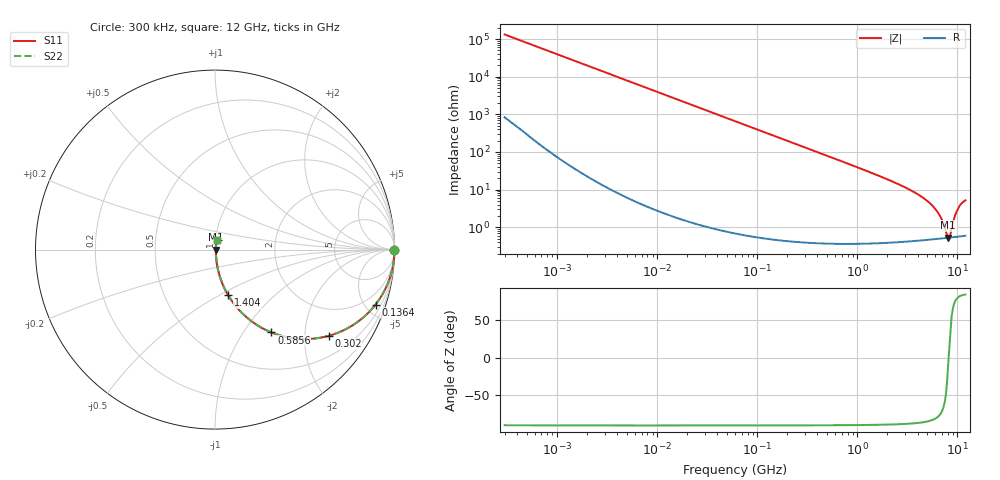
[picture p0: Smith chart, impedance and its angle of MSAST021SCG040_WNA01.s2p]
! MSAST021SCG040_WNA01  S-PARAMETER MODEL  ( General Type )
! Model Generated by TAIYO YUDEN Corporation (http://www.ty-top.com)
! Version 2.0
! TAIYO YUDEN Control No. 181101
! Copyright(c) 2015 TAIYO YUDEN CO.,LTD. All Rights Reserved.
! Product Description (link to TY-COMPAS)
! https://ds.yuden.co.jp/TYCOMPAS/or/detail?pn=MSAST021SCG040BWNA01&u=M
! Products Name : Multilayer Ceramic Capacitors
! Characteristics :
!  Capacitance : 4 pF , Rated Voltage : 25V , TCC : CG / C0G
!  Case Size : 0.25 x 0.125 / 0.0098 x 0.0049 [mm/inch] , Thickness : 0.125 / 0.0049 [mm/inch]
!  (Conditions: Temperature = 25 degC , DC Bias Current/Voltage = 0A / 0V)
! External Node Assignments :
!  1  o---| |---o  2
! GND o---------o GND
! Frequency Range : 0.3MHz  -  12000MHz  [ 401 STEP ]
# MHz S RI R 50
! Freq[MHz].  S11 Real  S11 Imag  S21 Real  S21 Imag  S12 Real  S12 Imag  S22 Real  S22 Imag
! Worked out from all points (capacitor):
!   401 points, 300 kHz to 12 GHz, reference 50 ohm
!   read as one part in series: C = 4 pF near 316.3 kHz
!   lowest |Z| = 534 mohm at 8.065 GHz (marker M1)
!   series resonance near 8.167 GHz, so ESL is about 95 pH
!   S11 on the Smith chart (normalised r, x): 300 kHz: open; 136.4 MHz: 1.01, -5.83; 302 MHz: 1.01, -2.63; 585.6 MHz: 1.01, -1.35; 1.404 GHz: 1.01, -0.55; 12 GHz: 1.01, +0.10
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0.3  1 -0.000754  5.31e-06 0.000754  5.31e-06 0.000754  1 -0.000754
1.769972  1 -0.00445  2.52e-05 0.00445  2.52e-05 0.00445  1 -0.00445
10.44266  0.9993 -0.0262  0.000706 0.0262  0.000706 0.0262  0.9993 -0.0262
60  0.9776 -0.1474  0.0224 0.1474  0.0224 0.1474  0.9776 -0.1474
136.3989  0.8944 -0.3065  0.1056 0.3065  0.1056 0.3065  0.8944 -0.3065
301.9711  0.6335 -0.4804  0.3665 0.4804  0.3665 0.4804  0.6335 -0.4804
353.9943  0.5571 -0.495  0.4429 0.495  0.4429 0.495  0.5571 -0.495
585.5907  0.3145 -0.4617  0.6855 0.4617  0.6855 0.4617  0.3145 -0.4617
894.6982  0.1638 -0.366  0.8362 0.366  0.8362 0.366  0.1638 -0.366
1403.667  0.0733 -0.2539  0.9267 0.2539  0.9267 0.2539  0.0733 -0.2539
2088.533  0.0342 -0.1712  0.9658 0.1712  0.9658 0.1712  0.0342 -0.1712
3642.919  0.0118 -0.086  0.9882 0.086  0.9882 0.086  0.0118 -0.086
5278.635  0.00654 -0.0432  0.9935 0.0432  0.9935 0.0432  0.00654 -0.0432
6524.734  0.0054 -0.0216  0.9946 0.0216  0.9946 0.0216  0.0054 -0.0216
7064.448  0.00523 -0.0138  0.9948 0.0138  0.9948 0.0138  0.00523 -0.0138
7854.144  0.00521 -0.00351  0.9948 0.00351  0.9948 0.00351  0.00521 -0.00351
8064.993  0.00524 -0.000921  0.9948 0.000921  0.9948 0.000921  0.00524 -0.000921
8503.825  0.00533 0.00349  0.9947 -0.00349  0.9947 -0.00349  0.00533 0.00349
9454.42  0.00587 0.0196  0.9941 -0.0196  0.9941 -0.0196  0.00587 0.0196
9968.853  0.00633 0.0273  0.9937 -0.0273  0.9937 -0.0273  0.00633 0.0273
10793.46  0.00733 0.0401  0.9927 -0.0401  0.9927 -0.0401  0.00733 0.0401
12000  0.00852 0.0509  0.9915 -0.0509  0.9915 -0.0509  0.00852 0.0509
